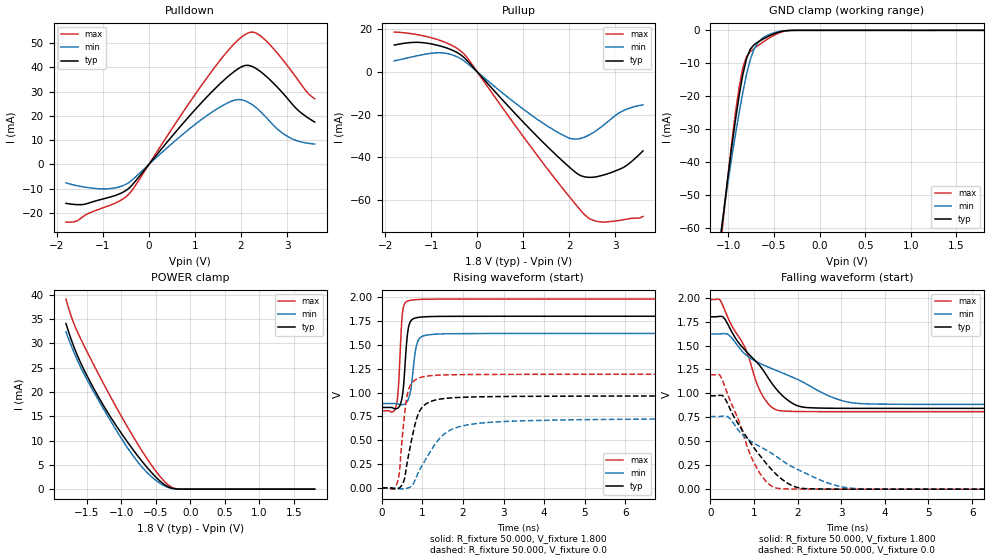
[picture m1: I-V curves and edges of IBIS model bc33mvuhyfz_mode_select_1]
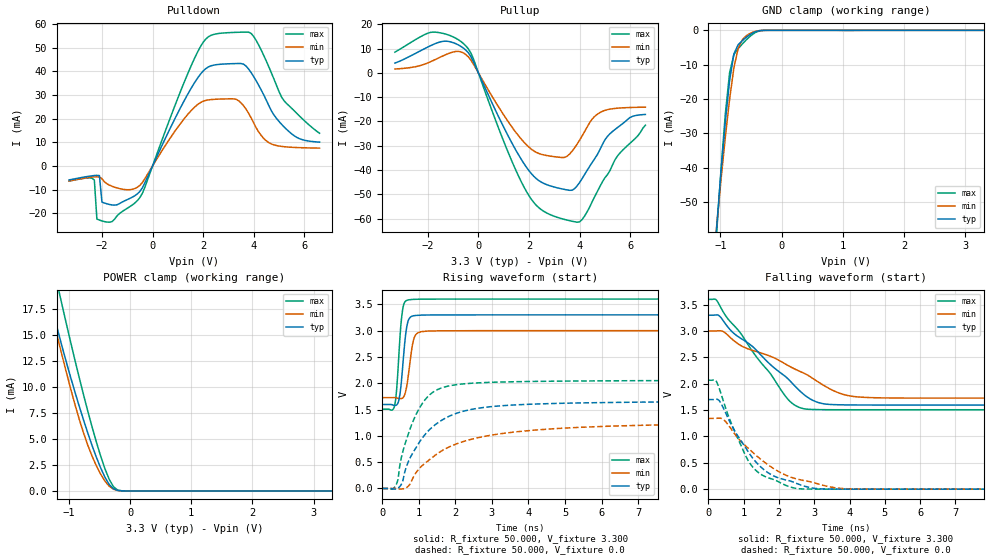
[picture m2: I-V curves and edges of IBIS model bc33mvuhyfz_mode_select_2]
|Texas Instruments Incorporated
|DP83825 Robust, Low Power 10/100 Ethernet Physical Layer Transceiver
[IBIS ver]   4.2
[File name]  dp83825.ibs
[File Rev]   1.0
[Date]   08/23/2018
[Source]
| Texas Instruments Incorporated.
| Analog-eLab Design Center, HPA
| 12500 TI Blvd
| Dallas, TX -75243
[Notes]   Revision History:
| Rev 1.0: 08/23/2018
| - Initial version of the model
| - Warnings regarding combined Non-monotonicity of various models
|   have been reviewed and considered minor and can be ignored.
| - Model names with a trailing _1 contain the model for
|   1.8V operation. Model names with a trailing _2 contain the model
|   for 3.3V operation.
| - C_comp although listed in numerical order of value are
|   obtained from varying PVT conditions. For PVT conditions for
|   each specific value refer the buffer description under
|   respective [Model]. IBIS model user is responsible for using
|   appropriate C_comp to simulate for Signal Integrity.
[Disclaimer]
| This model is designed as an aid for customers of Texas Instruments.
| TI and its licensors and suppliers make no warranties, either expressed
| or implied, with respect to this  model, including the warranties of
| merchantability or fitness for a particular purpose. The model is
| provided solely on an "as is" basis. The entire risk as to its quality
| and performance is with the customer.
| This model is subject to change without notice. Texas Instruments
| Incorporated is not responsible for updating this model.
[Copyright]
(C) Copyright 2018 Texas Instruments Incorporated.All rights reserved.
|  Component DP83825S 24-pin QFP
|  Part # DP83825S
[Component]   DP83825S
[Manufacturer] TI
[Package]   |24 QFP
| variable   typ   min   max
R_pkg   0.05   0.04   0.06
L_pkg   1.0nH   0.8nH   1.2nH
C_pkg   0.2pF   0.16pF   0.24pF
[Pin]  signal_name   model_name   R_pin   L_pin   C_pin
1   TX_EN   bc33mvuhyfz_mode_select   NA   NA   NA
2   Clkout50Mhz/LED_2   bc33mvuhyfz_mode_select   NA   NA   NA
3   INT/PWRDN   bc33mvuhyfz_mode_select   NA   NA   NA
4   LED_0_3V3   bc33mvuhyfz_mode_select   NA   NA   NA
5   RST   bc33mvuhyfz_mode_select   NA   NA   NA
6   VDDA3.3   power   NA   NA   NA
7   RD_M   nc   NA   NA   NA
8   RD_P   nc   NA   NA   NA
9   GND   gnd   NA   NA   NA
10   TD_M   nc   NA   NA   NA
11   TD_P   nc   NA   NA   NA
12   XO   nc   NA   NA   NA
13   XI/50MhzIn   nc   NA   NA   NA
14   RBIAS   nc   NA   NA   NA
15   MDIO   bc33mvuhyfz_mode_select   NA   NA   NA
16   MDC   bc33mvuhyfz_mode_select   NA   NA   NA
17   RX_D1   bc33mvuhyfz_mode_select   NA   NA   NA
18   RX_D0   bc33mvuhyfz_mode_select   NA   NA   NA
19   VDDIO   power   NA   NA   NA
20   CRS_DV   bc33mvuhyfz_mode_select   NA   NA   NA
21   GND   gnd   NA   NA   NA
22   RX_ER   bc33mvuhyfz_mode_select   NA   NA   NA
23   TX_D0   bc33mvuhyfz_mode_select   NA   NA   NA
24   TX_D1   bc33mvuhyfz_mode_select   NA   NA   NA
[Model Selector] bc33mvuhyfz_mode_select
bc33mvuhyfz_mode_select_1  1.8V operation
bc33mvuhyfz_mode_select_2  3.3V operation
| Models and submodels in the file (2): bc33mvuhyfz_mode_select_1 (I/O), bc33mvuhyfz_mode_select_2 (I/O)
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|   Model bc33mvuhyfz_mode_select_1
[Model] bc33mvuhyfz_mode_select_1
Model_type I/O
Polarity   Non-Inverting
Enable   Active-Low
Vinl =  0.330V
Vinh =  0.770V
Vmeas =  0.900V
C_comp   0.449pF   0.431pF   0.503pF
[Model Spec]
Vinh   0.770V   0.693V   0.847V
Vinl   0.330V   0.297V   0.363V
Vmeas   0.900V   0.810V   0.990V
[Temperature Range]   25.000   0.125k   -40.000
[Voltage Range]   1.800V   1.620V   1.980V
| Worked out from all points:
|   slope of the pulldown table from 0 to 0.27 V, typ, clamps not added: 42.9 ohm
|   slope of the pullup table from 0 to 0.27 V, typ, clamps not added: 41.5 ohm
|   GND clamp passes 1 mA (typ) near -0.50 V on its own axis
|   POWER clamp passes 1 mA (typ) near -0.38 V on its own axis
|   rising waveform, R_fixture 50.000, V_fixture 1.800: 20-80 % time 105ps typ, 129ps min, 84.5ps max; typ from 0.844 V to 1.8 V
|   rising waveform, R_fixture 50.000, V_fixture 0.0: 20-80 % time 301ps typ, 738ps min, 170ps max; typ from 0 V to 0.97 V
|   falling waveform, R_fixture 50.000, V_fixture 1.800: 20-80 % time 998ps typ, 1.79ns min, 673ps max; typ from 1.8 V to 0.844 V
|   falling waveform, R_fixture 50.000, V_fixture 0.0: 20-80 % time 910ps typ, 1.59ns min, 617ps max; typ from 0.975 V to 0 V
[Pulldown]
|Voltage   I(typ)   I(min)   I(max)
-1.8V     -16mA      -7.545mA   -23.69mA
-1.44V    -16.49mA   -9.163mA   -21.57mA
-960mV    -14.01mA   -10.04mA   -17.58mA
-420mV    -9.558mA   -7.246mA   -11.92mA
660mV     15.11mA    11.18mA    19.21mA
1.38V     30.11mA    21.65mA    38.72mA
1.86V     38.33mA    26.46mA    49.79mA
2.16V     40.77mA    25.55mA    54.16mA
2.34V     39.34mA    23.22mA    53.94mA
2.58V     35.71mA    18.69mA    50.23mA
3.06V     26.02mA    11.04mA    39.36mA
3.6V      17.46mA    8.405mA    27.07mA
[Pullup]
|Voltage   I(typ)   I(min)   I(max)
-1.8V     12.49mA    5.082mA    18.54mA
-1.32V    13.77mA    7.412mA    17.43mA
-840mV    12.26mA    8.901mA    14.89mA
-540mV    10.11mA    7.891mA    12.22mA
-300mV    6.96mA     5.347mA    8.626mA
1.5V      -34.4mA    -24.98mA   -44.59mA
1.98V     -44.09mA   -30.78mA   -57.74mA
2.28V     -48.73mA   -30.9mA    -65.5mA
2.58V     -49.03mA   -27.51mA   -69.69mA
3.06V     -45.76mA   -19.48mA   -69.47mA
3.3V      -42.81mA   -17.02mA   -68.57mA
3.6V      -36.92mA   -15.42mA   -67.55mA
[GND_clamp]
|Voltage   I(typ)   I(min)   I(max)
-1.8V     -249.2mA   -226.4mA   -267.3mA
-1.08V    -61.63mA   -60.64mA   -63.68mA
-1.04V    -52.25mA   -52.75mA   -53.14mA
-960mV    -34.62mA   -37.95mA   -33.2mA
-920mV    -26.62mA   -31.06mA   -24.33mA
-880mV    -19.37mA   -24.56mA   -16.8mA
-840mV    -13.13mA   -18.54mA   -11.12mA
-800mV    -8.427mA   -13.21mA   -7.86mA
-720mV    -4.403mA   -5.765mA   -5.523mA
-600mV    -2.351mA   -1.9mA     -3.166mA
-320mV    -27.6uA    -28.66uA   -42.52uA
1.8V      0A         0A         -51.48nA
[POWER_clamp]
|Voltage   I(typ)   I(min)   I(max)
-1.8V     34.07mA    32.37mA    39.11mA
-1.68V    29.08mA    28mA       33.87mA
-1.48V    22.91mA    22.12mA    27.86mA
-1.24V    16.8mA     16.12mA    21.27mA
-960mV    10.71mA    9.604mA    14.05mA
-800mV    7.575mA    6.321mA    10.18mA
-640mV    4.702mA    3.632mA    6.575mA
-480mV    2.215mA    1.613mA    3.358mA
-320mV    474.9uA    349.3uA    876.9uA
-240mV    107.7uA    94uA       214.8uA
-120mV    4.21uA     6.678uA    6.349uA
1.8V      0A         0A         0A
[Ramp]
| variable   typ   min   max
dV/dt_r   0.582/0.301n   0.443/0.735n   0.716/0.169n
dV/dt_f   0.574/0.997n   0.441/1.787n   0.702/0.672n
R_load = 50.000
[Rising Waveform]
R_fixture= 50.000
V_fixture= 1.800
V_fixture_min= 1.620
V_fixture_max= 1.980
|time   V(typ)   V(min)   V(max)
0s        843.8mV    885mV      809.4mV
346ps     830.1mV    885mV      850.2mV
398ps     838.2mV    879.8mV    994.8mV
451ps     870.7mV    873.2mV    1.419V
540ps     1.097V     875.7mV    1.908V
646ps     1.657V     922.8mV    1.96V
803ps     1.778V     1.362V     1.973V
942ps     1.79V      1.573V     1.976V
1.556ns   1.799V     1.616V     1.98V
30ns      1.8V       1.62V      1.98V
[Rising Waveform]
R_fixture= 50.000
V_fixture= 0.0
V_fixture_min= 0.0
V_fixture_max= 0.0
|time   V(typ)   V(min)   V(max)
0s        74.92uV    71.12uV    79.05uV
270ps     -3.458mV   -588.1nV   -10.39mV
402ps     -5.779mV   -5.394mV   85.92mV
581ps     148.1mV    -6.893mV   850mV
693ps     420.1mV    8.237mV    1.067V
904ps     782.5mV    164.8mV    1.151V
1.184ns   903.3mV    373.4mV    1.176V
1.834ns   947.3mV    632.4mV    1.187V
3.373ns   959.9mV    702.9mV    1.191V
30ns      969.6mV    738.6mV    1.194V
[Falling Waveform]
R_fixture= 50.000
V_fixture= 1.800
V_fixture_min= 1.620
V_fixture_max= 1.980
|time   V(typ)   V(min)   V(max)
0s        1.8V       1.62V      1.98V
252ps     1.804V     1.623V     1.954V
437ps     1.693V     1.606V     1.76V
799ps     1.451V     1.411V     1.477V
1.239ns   1.225V     1.292V     947.6mV
1.659ns   974.6mV    1.213V     817mV
2.106ns   858.1mV    1.122V     810.3mV
2.882ns   844.6mV    944.4mV    809.4mV
3.563ns   843.8mV    891.1mV    809.3mV
30ns      843.7mV    885mV      809.3mV
[Falling Waveform]
R_fixture= 50.000
V_fixture= 0.0
V_fixture_min= 0.0
V_fixture_max= 0.0
|time   V(typ)   V(min)   V(max)
0s        975.1mV    758.4mV    1.194V
251ps     979.7mV    761.2mV    1.167V
416ps     877.5mV    751.1mV    971.5mV
751ps     602.5mV    562.8mV    584.8mV
1.102ns   372.3mV    453.9mV    192.8mV
1.335ns   241.2mV    394.4mV    56.57mV
1.565ns   133.4mV    325.4mV    7.963mV
2.072ns   10.3mV     190.6mV    810.5uV
3.4ns     91.16uV    4.962mV    6.446uV
30ns      905.2nV    5.027uV    479.5nV
|   Model bc33mvuhyfz_mode_select_2
[Model] bc33mvuhyfz_mode_select_2
Model_type I/O
Polarity   Non-Inverting
Enable   Active-Low
Vinl =  0.330V
Vinh =  0.770V
Vmeas =  1.650V
C_comp   0.419pF   0.391pF   0.491pF
[Model Spec]
Vinh   0.770V   0.693V   0.847V
Vinl   0.330V   0.297V   0.363V
Vmeas   1.650V   1.500V   1.800V
[Temperature Range]   25.000   0.125k   -40.000
[Voltage Range]   3.300V   3.000V   3.600V
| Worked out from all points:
|   slope of the pulldown table from 0 to 0.495 V, typ, clamps not added: 43.3 ohm
|   slope of the pullup table from 0 to 0.495 V, typ, clamps not added: 43.5 ohm
|   GND clamp passes 1 mA (typ) near -0.50 V on its own axis
|   POWER clamp passes 1 mA (typ) near -0.38 V on its own axis
|   rising waveform, R_fixture 50.000, V_fixture 3.300: 20-80 % time 137ps typ, 153ps min, 122ps max; typ from 1.6 V to 3.3 V
|   rising waveform, R_fixture 50.000, V_fixture 0.0: 20-80 % time 1.11ns typ, 2.25ns min, 654ps max; typ from 0 V to 1.67 V
|   falling waveform, R_fixture 50.000, V_fixture 3.300: 20-80 % time 1.76ns typ, 2.37ns min, 1.4ns max; typ from 3.3 V to 1.6 V
|   falling waveform, R_fixture 50.000, V_fixture 0.0: 20-80 % time 1.08ns typ, 1.46ns min, 830ps max; typ from 1.7 V to 0 V
[Pulldown]
|Voltage   I(typ)   I(min)   I(max)
-3.3V     -5.902mA   -6.343mA   -6.394mA
-2.3V     -4.031mA   -4.586mA   -5.953mA
-2.2V     -3.964mA   -4.557mA   -22.41mA
-2.1V     -4.064mA   -4.682mA   -22.84mA
-2V       -15.26mA   -5.39mA    -23.2mA
-600mV    -11.78mA   -8.982mA   -14.62mA
1.7V      35.86mA    25.23mA    46.42mA
2.5V      42.76mA    28.19mA    55.78mA
3.3V      43.27mA    28.15mA    56.45mA
3.9V      39.39mA    20.22mA    55.95mA
5.2V      16.48mA    8.147mA    27.53mA
6.6V      10.07mA    7.548mA    13.82mA
[Pullup]
|Voltage   I(typ)   I(min)   I(max)
-3.3V     4.03mA     1.576mA    8.509mA
-1.8V     11.61mA    5.01mA     16.78mA
-1.2V     12.97mA    7.876mA    15.65mA
-500mV    9.388mA    7.557mA    11.15mA
1.9V      -38.88mA   -29.62mA   -48.86mA
2.5V      -45.08mA   -33.58mA   -56.42mA
3.3V      -47.77mA   -34.86mA   -60.06mA
3.7V      -48.34mA   -32.3mA    -61.08mA
4.1V      -43.52mA   -25.96mA   -60.4mA
4.6V      -35.28mA   -17.89mA   -50.92mA
5.2V      -25.07mA   -14.94mA   -40.25mA
6.6V      -17.12mA   -14.12mA   -21.55mA
[GND_clamp]
|Voltage   I(typ)   I(min)   I(max)
-3.3V     -664.5mA   -595.8mA   -721.5mA
-1.06V    -56.9mA    -56.66mA   -58.38mA
-990mV    -41.02mA   -43.34mA   -40.43mA
-920mV    -26.62mA   -31.06mA   -24.33mA
-850mV    -14.57mA   -19.99mA   -12.34mA
-780mV    -6.819mA   -10.88mA   -7.02mA
-710mV    -4.182mA   -5.191mA   -5.314mA
-640mV    -2.958mA   -2.675mA   -3.918mA
-500mV    -1.041mA   -738.5uA   -1.5mA
-430mV    -397.4uA   -278.5uA   -631.7uA
-290mV    -11.03uA   -14.09uA   -14.3uA
3.3V      0A         0A         -53.46nA
[POWER_clamp]
|Voltage   I(typ)   I(min)   I(max)
-3.3V     223.9mA    167.2mA    277.8mA
-1.39V    20.51mA    19.81mA    25.35mA
-1.32V    18.74mA    18.07mA    23.43mA
-1.18V    15.42mA    14.67mA    19.68mA
-1.11V    13.86mA    13.01mA    17.85mA
-900mV    9.507mA    8.318mA    12.57mA
-690mV    5.567mA    4.398mA    7.668mA
-550mV    3.242mA    2.417mA    4.704mA
-410mV    1.322mA    948.1uA    2.142mA
-270mV    202.1uA    161.6uA    399.8uA
-60mV     511.1nA    1.232uA    554.9nA
3.3V      0A         0A         0A
[Ramp]
| variable   typ   min   max
dV/dt_r   1.005/1.110n   0.772/2.244n   1.237/0.654n
dV/dt_f   1.023/1.763n   0.764/2.367n   1.256/1.399n
R_load = 50.000
[Rising Waveform]
R_fixture= 50.000
V_fixture= 3.300
V_fixture_min= 3.000
V_fixture_max= 3.600
|time   V(typ)   V(min)   V(max)
0s        1.596V     1.726V     1.507V
325ps     1.578V     1.727V     1.548V
387ps     1.586V     1.723V     1.85V
439ps     1.648V     1.711V     2.385V
563ps     2.372V     1.724V     3.429V
666ps     3.064V     1.937V     3.574V
786ps     3.265V     2.558V     3.591V
943ps     3.29V      2.943V     3.596V
1.497ns   3.299V     2.996V     3.599V
30ns      3.3V       3V         3.6V
[Rising Waveform]
R_fixture= 50.000
V_fixture= 0.0
V_fixture_min= 0.0
V_fixture_max= 0.0
|time   V(typ)   V(min)   V(max)
0s        75.04uV    71.33uV    79.21uV
373ps     -10.02mV   -1.374mV   64.87mV
532ps     94.57mV    -9.335mV   622.5mV
632ps     357.8mV    5.647mV    869.6mV
1.125ns   988.2mV    455.5mV    1.647V
1.527ns   1.252V     671.9mV    1.885V
2.137ns   1.452V     874.2mV    1.982V
3.695ns   1.591V     1.079V     2.03V
7.015ns   1.64V      1.199V     2.049V
30ns      1.674V     1.286V     2.061V
[Falling Waveform]
R_fixture= 50.000
V_fixture= 3.300
V_fixture_min= 3.000
V_fixture_max= 3.600
|time   V(typ)   V(min)   V(max)
0s        3.3V       3V         3.6V
229ps     3.305V     3.001V     3.59V
430ps     3.19V      2.989V     3.357V
1.019ns   2.82V      2.691V     2.857V
2.251ns   2.098V     2.349V     1.71V
2.78ns    1.758V     2.177V     1.519V
3.159ns   1.635V     2.014V     1.509V
3.699ns   1.601V     1.825V     1.507V
4.659ns   1.596V     1.735V     1.506V
30ns      1.596V     1.726V     1.506V
[Falling Waveform]
R_fixture= 50.000
V_fixture= 0.0
V_fixture_min= 0.0
V_fixture_max= 0.0
|time   V(typ)   V(min)   V(max)
0s        1.7V       1.342V     2.066V
245ps     1.705V     1.345V     2.026V
437ps     1.528V     1.319V     1.656V
739ps     1.116V     1.059V     1.114V
1.06ns    786.2mV    819.4mV    633.6mV
1.269ns   581.2mV    693.5mV    413.1mV
1.781ns   276.4mV    422.2mV    197.4mV
2.607ns   82.07mV    177.2mV    6.168mV
4.093ns   390.3uV    3.815mV    21.11uV
30ns      933.7nV    5.19uV     513.7nV
